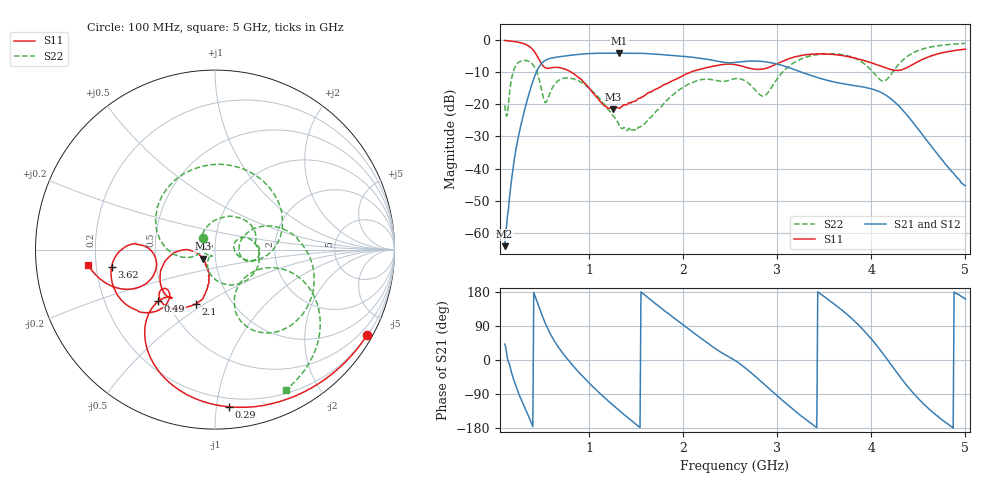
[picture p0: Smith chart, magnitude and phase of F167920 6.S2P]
!  2-Port S-parameters saved by WinCal
! VAR MeasName=S-Parameters (CALIBRATED_DATA) read from VNA (N5242A)
! VAR MeasDate=2016-11-22 9:53:47
! VAR NAME=F167920 6
! VAR FILENAME=F167920 6.S2P
! VAR DATE=2016-11-22 9:53:47
! VAR PHYS_PORTS=1,2
# Hz S DB R 50
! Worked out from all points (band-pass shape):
!   491 points, 100 MHz to 5 GHz, reference 50 ohm
!   highest |S21| = -4.15 dB at 1.32 GHz (marker M1); lowest = -64.0 dB at 100 MHz (marker M2)
!   |S21| within 3 dB of the highest: 501.6 MHz to 2.47 GHz (1.969 GHz wide, 132 % of centre); 2.517 GHz to 2.933 GHz (416.3 MHz wide, 15.3 % of centre)
!   lowest |S11| = -21.5 dB at 1.25 GHz (marker M3), VSWR 1.18, Z = 43.4 - j4.35 ohm
!   |S11| at or under -10 dB: 804.2 MHz to 2.085 GHz (1.28 GHz wide, 88.6 % of centre)
!   |S22| runs from -28.3 to -1.2 dB; largest |S21 - S12| = 0.0018
!   S11 on the Smith chart (normalised r, x): 100 MHz: 0.22, -3.82; 290 MHz: 0.14, -1.08; 490 MHz: 0.45, -0.32; 2.1 GHz: 0.68, -0.46; 3.62 GHz: 0.26, -0.08; 5 GHz: 0.17, -0.06
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1e8  -0.25 -29.3  -64.01 42.1  -65.01 28.9  -20.40 135.3
1.3e8  -0.33 -37.9  -54.73 4.4  -54.12 1.4  -23.14 -178.0
2.1e8  -0.62 -60.9  -35.82 -61.2  -35.90 -61.0  -8.53 152.1
2.9e8  -1.12 -84.9  -24.42 -112.1  -24.40 -111.9  -6.49 92.5
3.9e8  -2.78 -117.7  -13.84 -169.3  -13.82 -169.3  -7.39 29.7
4.9e8  -7.38 -137.6  -7.50 123.4  -7.49 123.4  -15.14 -18.5
5.4e8  -8.79 -133.3  -6.32 92.8  -6.31 92.8  -19.48 9.9
7e8  -8.76 -144.8  -5.23 24.2  -5.22 24.2  -12.22 -3.0
9.2e8  -12.44 -174.6  -4.45 -40.2  -4.44 -40.3  -13.31 -66.4
1.25e9  -21.46 -143.9  -4.18 -118.5  -4.18 -118.6  -23.59 -123.7
1.32e9  -21.29 -132.1  -4.15 -133.1  -4.15 -133.1  -26.88 -128.0
1.49e9  -18.96 -112.1  -4.23 -168.1  -4.23 -168.1  -27.89 -124.3
1.74e9  -14.87 -101.2  -4.57 141.8  -4.56 141.8  -21.43 155.7
2.1e9  -9.81 -109.6  -5.46 73.6  -5.44 73.6  -13.26 55.9
2.55e9  -7.73 -138.9  -7.05 -1.1  -7.04 -1.2  -12.09 0.0
2.93e9  -8.35 -132.4  -7.13 -79.3  -7.11 -79.4  -15.16 24.3
3.37e9  -4.48 -153.5  -11.21 -169.3  -11.18 -169.5  -4.92 -13.6
3.62e9  -4.66 -170.3  -13.21 144.8  -13.21 144.6  -4.42 -42.1
3.97e9  -6.91 175.8  -15.02 63.9  -15.03 63.8  -8.62 -71.7
4.19e9  -9.12 -177.9  -17.95 -5.6  -17.94 -5.8  -11.50 -24.8
4.51e9  -6.60 -153.6  -28.19 -104.5  -28.20 -104.7  -3.24 -32.0
5e9  -2.95 -173.1  -45.22 160.6  -45.72 161.1  -1.15 -63.3
